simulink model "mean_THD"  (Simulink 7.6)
settings: Solver=ode23tb  StartTime=0.0  StopTime=0.2  RelTol=1e-3
InitFcn:
  | T=1/60;
  | Arms=100;
StopFcn:
  | close all
  | load Va_MeanVa.mat
  | subplot 211
  | plot(x(1,:),x(2,:))
  | grid
  | title('Tension phase A')
  | 
  | subplot 212
  | plot(x(1,:),x(3,:))
  | axis([0 0.2 -15 10])
  | grid
  | title('Moyenne tension phase A')
  | xlabel('temps')
  | 
  | 
  | figure
  | load THD_RMS.mat
  | subplot 211
  | plot(y(1,:),y(2,:))
  | grid
  | title('Taux de distorsion THD de la phase B')
  | axis([0 0.2 -0.2 1])
  | 
  | subplot 212
  | plot(y(1,:),y(3,:))
  | axis([0 0.2 0 80])
  | grid
  | title('Valeur efficace de la phase B')
  | xlabel('temps')
  | 
  | delete *.mat
libraries: powerlib x8, powerlib_extras x3

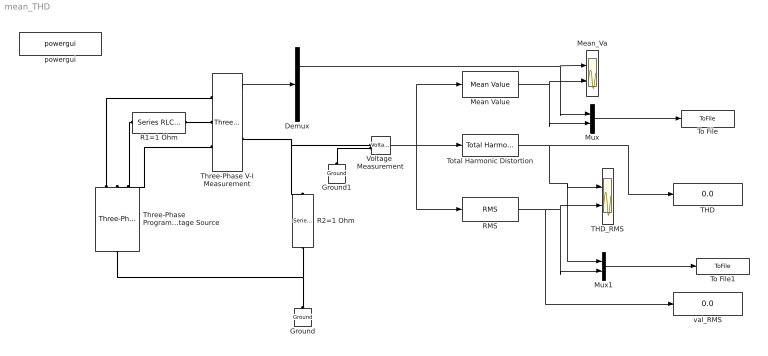
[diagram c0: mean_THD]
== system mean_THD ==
  Demux : Demux  Outputs=3
  Ground : powerlib/Elements/Ground  DialogController=POWERSYS.PowerSysDialog  PhysicalDomain=powersysdomain  SubClassName=unknown  LeftPortType=p1  RightPortType=p1  LConnTagsString=a
  Ground1 : powerlib/Elements/Ground  DialogController=POWERSYS.PowerSysDialog  PhysicalDomain=powersysdomain  SubClassName=unknown  LeftPortType=p1  RightPortType=p1  LConnTagsString=a
  Mean Value : powerlib_extras/Measurements/Mean Value  DialogController=POWERSYS.PowerSysDialog  SystemSampleTime=-1  Period=T
  Mean_Va : Scope  NumInputPorts=2
  Mux : Mux  Inputs=2
  Mux1 : Mux  Inputs=2
  R1=1 Ohm : powerlib/Elements/Series RLC Branch  DialogController=POWERSYS.PowerSysDialog  PhysicalDomain=powersysdomain  SubClassName=unknown  LeftPortType=p1  RightPortType=p1  LConnTagsString=__new0  RConnTagsString=__new0  BranchType=R  Resistance=1  Inductance=1e-3  SetiL0=off  InitialCurrent=0  Capacitance=1e-6  Setx0=off  InitialVoltage=0  Measurements=None
  R2=1 Ohm : powerlib/Elements/Series RLC Branch  DialogController=POWERSYS.PowerSysDialog  PhysicalDomain=powersysdomain  SubClassName=unknown  LeftPortType=p1  RightPortType=p1  LConnTagsString=__new0  RConnTagsString=__new0  BranchType=R  Resistance=1  Inductance=1e-3  SetiL0=off  InitialCurrent=0  Capacitance=1e-6  Setx0=off  InitialVoltage=0  Measurements=None
  RMS : powerlib_extras/Measurements/RMS  DialogController=POWERSYS.PowerSysDialog  SystemSampleTime=-1  f1=60
  THD : Display
  THD_RMS : Scope  NumInputPorts=2
  Three-Phase Programmable Voltage Source : powerlib/Electrical Sources/Three-Phase Programmable Voltage Source  DialogController=POWERSYS.PowerSysDialog  SystemSampleTime=-1  PositiveSequence="[Arms  0 1/T]"  VariationEntity=Amplitude  VariationType=Step  VariationStep=1  VariationRate=10  VariationMagnitude=0.3  VariationFrequency=2  VariationTiming="[0.06  0.14  0.2]"  VariationPhaseA=off  Amplitudes=[1 0.8 1.2 1.0]  TimeValues=[0 0.1 0.15 0.2]  HarmonicGeneration=on  HarmonicA="[3 0.2  -25 0]"  HarmonicB=[2 0.15 35 2]  Timing="[0.1  0.2]"
  Three-Phase V-I Measurement : powerlib/Measurements/Three-Phase V-I Measurement  DialogController=POWERSYS.PowerSysDialog  SystemSampleTime=-1  VoltageMeasurement=phase-to-ground  SetLabelV=off  LabelV=V1  Vpu=on  VpuLL=off  CurrentMeasurement=yes  SetLabelI=off  LabelI=I1  Ipu=on  Pbase=10e6  Vbase=25e3  OutputType=Magnitude  PhasorSimulation=off  PSBequivalent=0
  To File : ToFile  Filename=Va_MeanVa  MatrixName=x
  To File1 : ToFile  Filename=THD_RMS  MatrixName=y
  Total Harmonic Distortion : powerlib_extras/Measurements/Total Harmonic Distortion  DialogController=POWERSYS.PowerSysDialog  SystemSampleTime=-1  f1=60
  Voltage  Measurement : powerlib/Measurements/Voltage Measurement  DialogController=POWERSYS.PowerSysDialog  SystemSampleTime=-1  PhasorSimulation=off  OutputType=Complex  PSBequivalent=0
  powergui : powerlib/powergui  Priority=2  SystemSampleTime=-1  SimulationMode=Discrete  SampleTime=50e-6  frequency=60  SPID=off  DisableSnubberDevices=off  DisableRonSwitches=off  DisableVfSwitches=off  SwTol=0  Interpol=off  frequencyindice=60  echomessages=off  HookPort=off  DisplayEquations=off  FunctionMessages=off  EnableUseOfTLC=off  x0status=blocks  RestoreLinks=warning  ResistiveCurrentMeasurement=off  Frange=[0:2:500]  Ylog=off  Xlog=off  ShowGrid=off  save=off  variable=ZData  ZoomFFT=on  StartTime=0.0  cycles=1  DisplayStyle=off  fundamental=60  FreqAxis=off  MaxFrequency=1000  frequencyindicesteady=1  RmsSteady=1  display=off  Ts=0  methode=off
  val_RMS : Display
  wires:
  Voltage  Measurement/1 -> Total Harmonic Distortion/1, Mean Value/1, RMS/1
  Three-Phase V-I Measurement/1 -> Demux/1
  Mean Value/1 -> Mean_Va/2, Mux/2
  Demux/1 -> Mean_Va/1, Mux/1
  Total Harmonic Distortion/1 -> THD/1, THD_RMS/1, Mux1/1
  RMS/1 -> val_RMS/1, THD_RMS/2, Mux1/2
  Mux/1 -> To File/1
  Mux1/1 -> To File1/1
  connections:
  R2=1 Ohm/RConn1 -- Ground/LConn1 -- Three-Phase Programmable Voltage Source/LConn1
  R1=1 Ohm/LConn1 -- Three-Phase Programmable Voltage Source/RConn2
  R1=1 Ohm/RConn1 -- Three-Phase V-I Measurement/LConn2
  Three-Phase Programmable Voltage Source/RConn1 -- Three-Phase V-I Measurement/LConn1
  Three-Phase V-I Measurement/LConn3 -- Three-Phase Programmable Voltage Source/RConn3
  Three-Phase V-I Measurement/RConn2 -- R2=1 Ohm/LConn1 -- Voltage  Measurement/LConn1
  Ground1/LConn1 -- Voltage  Measurement/LConn2
